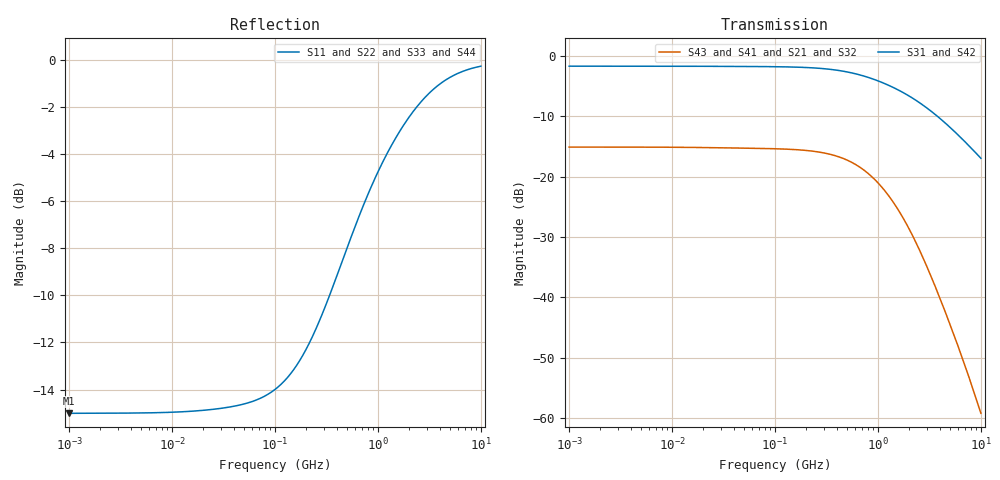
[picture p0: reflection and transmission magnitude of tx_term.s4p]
! Created Thu Apr 13 14:36:16 2017
# hz S ma R 50
! 4 Port Network Data from SP1.SP block
! freq  magS11  angS11  magS12  angS12  magS13  angS13  magS14  angS14
!  magS21  angS21  magS22  angS22  magS23  angS23  magS24  angS24
!  magS31  angS31  magS32  angS32  magS33  angS33  magS34  angS34
!  magS41  angS41  magS42  angS42  magS43  angS43  magS44  angS44
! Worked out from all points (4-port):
!   801 points, 1 MHz to 10 GHz, reference 50 ohm
!   strongest paths, dB at 1 MHz, 10 MHz, 100 MHz, 1 GHz, 10 GHz:
!     S31: -1.7, -1.7, -1.8, -4.1, -17.0
!     S42: -1.7, -1.7, -1.8, -4.1, -17.0
!     S43: -15.1, -15.1, -15.4, -21.0, -59.2
!     S41: -15.1, -15.1, -15.4, -21.0, -59.2
!     S21: -15.1, -15.1, -15.4, -21.0, -59.2
!     S32: -15.1, -15.1, -15.4, -21.0, -59.2
!   lowest |S11| = -15.0 dB at 1 MHz (marker M1), VSWR 1.43, Z = 34.9 - j0.0641 ohm
!   |S11| at or under -10 dB: start of sweep to 338.8 MHz
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1000000  0.1776 -179.7  0.1757 -0.2  0.8224 -0.1  0.1757 -0.2
         0.1757 -0.2  0.1776 -179.7  0.1757 -0.2  0.8224 -0.1
         0.8224 -0.1  0.1757 -0.2  0.1776 -179.7  0.1757 -0.2
         0.1757 -0.2  0.8224 -0.1  0.1757 -0.2  0.1776 -179.7
9.225714e7  0.1971 -162.0  0.1705 -11.2  0.8148 -4.3  0.1705 -11.2
            0.1705 -11.2  0.1971 -162.0  0.1705 -11.2  0.8148 -4.3
            0.8148 -4.3  0.1705 -11.2  0.1971 -162.0  0.1705 -11.2
            0.1705 -11.2  0.8148 -4.3  0.1705 -11.2  0.1971 -162.0
6.456542e8  0.462 -141.3  0.1219 -66.7  0.7014 -24.3  0.1219 -66.7
            0.1219 -66.7  0.4619 -141.3  0.1219 -66.7  0.7014 -24.3
            0.7014 -24.3  0.1219 -66.7  0.462 -141.3  0.1219 -66.7
            0.1219 -66.7  0.7014 -24.3  0.1219 -66.7  0.4619 -141.3
1.216186e9  0.6308 -147.3  0.07296 -104.4  0.5803 -36.0  0.07296 -104.4
            0.07296 -104.4  0.6308 -147.3  0.07296 -104.4  0.5803 -36.0
            0.5803 -36.0  0.07296 -104.4  0.6308 -147.3  0.07296 -104.4
            0.07296 -104.4  0.5803 -36.0  0.07296 -104.4  0.6308 -147.3
2.213095e9  0.7791 -154.9  0.03135 -143.0  0.4421 -48.3  0.03135 -143.0
            0.03135 -143.1  0.7791 -154.9  0.03135 -143.1  0.4421 -48.3
            0.4421 -48.3  0.03135 -143.0  0.7791 -154.9  0.03135 -143.0
            0.03135 -143.1  0.4421 -48.3  0.03135 -143.1  0.7791 -154.9
4.415704e9  0.9036 -164.0  0.007929 -180.0  0.2823 -62.2  0.007929 -180.0
            0.00792 -180.0  0.9036 -164.0  0.00792 -180.0  0.2823 -62.2
            0.2823 -62.2  0.007929 -180.0  0.9036 -164.0  0.007929 -180.0
            0.00792 -180.0  0.2823 -62.2  0.00792 -180.0  0.9036 -164.0
1e10  0.9708 -171.9  0.001092 150.1  0.1419 -74.1  0.001092 150.1
      0.001093 150.1  0.9708 -171.9  0.001093 150.1  0.1419 -74.1
      0.1419 -74.1  0.001092 150.1  0.9708 -171.9  0.001092 150.1
      0.001093 150.1  0.1419 -74.1  0.001093 150.1  0.9708 -171.9
